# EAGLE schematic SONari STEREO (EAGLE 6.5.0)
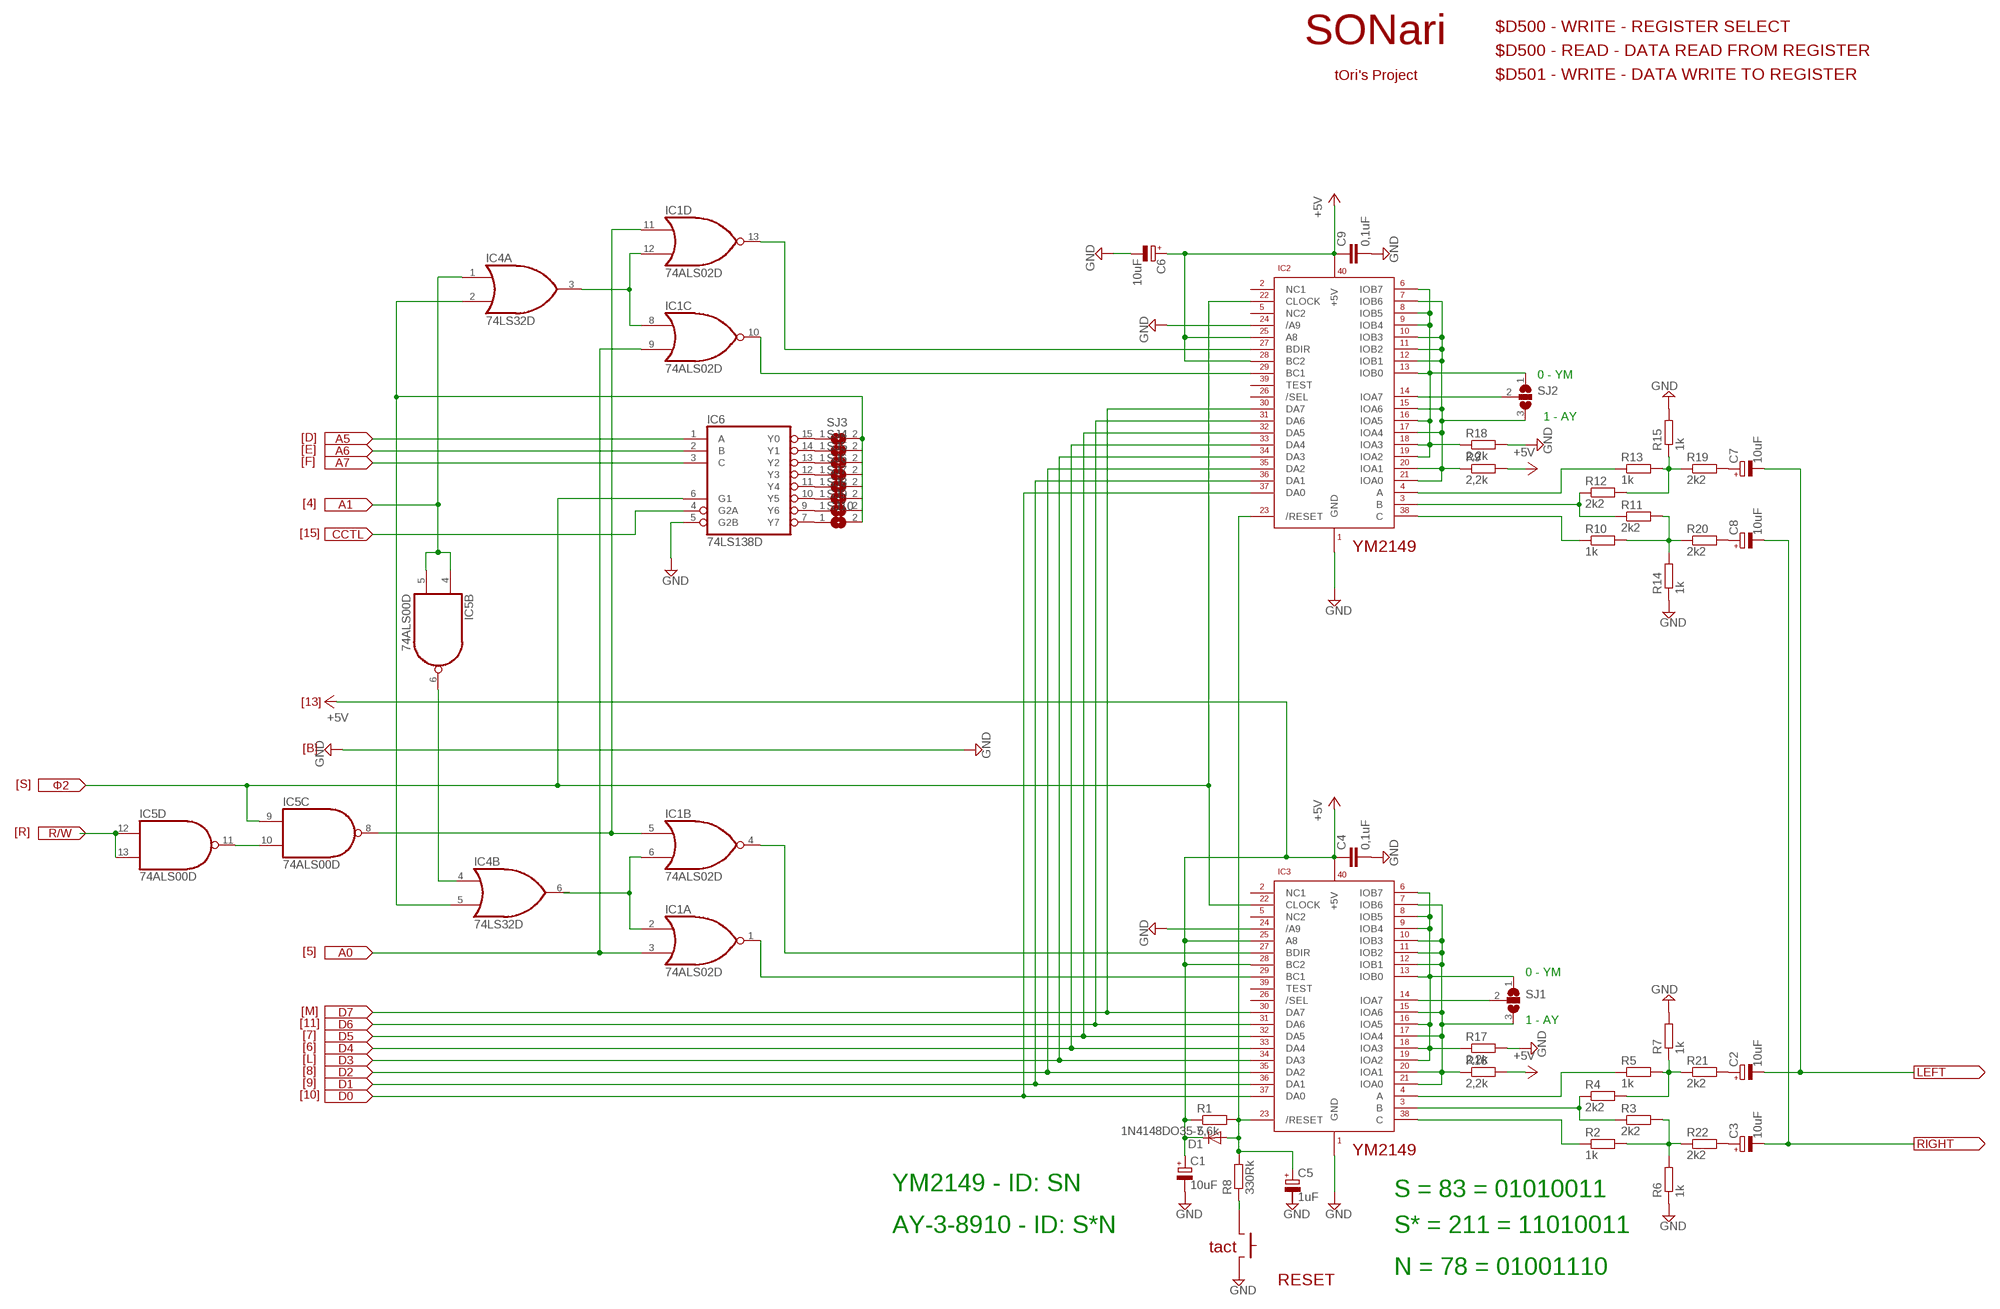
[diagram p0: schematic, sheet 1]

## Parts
C1  10uF  CPOL-EU085CS-1R  [085CS_1R]
C2  10uF  CPOL-EU085CS-1R  [085CS_1R]
C3  10uF  CPOL-EU085CS-1R  [085CS_1R]
C4  0,1uF  C-EUC0805  [C0805]
C5  1uF  CPOL-EU085CS-1R  [085CS_1R]
C6  10uF  CPOL-EU085CS-1R  [085CS_1R]
C7  10uF  CPOL-EU085CS-1R  [085CS_1R]
C8  10uF  CPOL-EU085CS-1R  [085CS_1R]
C9  0,1uF  C-EUC0805  [C0805]
D1  1N4148DO35-7  [DO35-7]
IC1  74ALS02D  [SO14]
IC2  YM2149  [YM2149]
IC3  YM2149  [YM2149]
IC4  74LS32D  [SO14]
IC5  74ALS00D  [SO14]
IC6  74LS138D  [SO16]
R1  5,6k  R-EU_R0805  [R0805]
R2  1k  R-EU_R0805  [R0805]
R3  2k2  R-EU_R0805  [R0805]
R4  2k2  R-EU_R0805  [R0805]
R5  1k  R-EU_R0805  [R0805]
R6  1k  R-EU_R0805  [R0805]
R7  1k  R-EU_R0805  [R0805]
R8  330Rk  R-EU_R0805  [R0805]
R9  2,2k  R-EU_R0805  [R0805]
R10  1k  R-EU_R0805  [R0805]
R11  2k2  R-EU_R0805  [R0805]
R12  2k2  R-EU_R0805  [R0805]
R13  1k  R-EU_R0805  [R0805]
R14  1k  R-EU_R0805  [R0805]
R15  1k  R-EU_R0805  [R0805]
R16  2,2k  R-EU_R0805  [R0805]
R17  2,2k  R-EU_R0805  [R0805]
R18  2,2k  R-EU_R0805  [R0805]
R19  2k2  R-EU_R0805  [R0805]
R20  2k2  R-EU_R0805  [R0805]
R21  2k2  R-EU_R0805  [R0805]
R22  2k2  R-EU_R0805  [R0805]
SJ1  SJ2W  [SJ_2]
SJ2  SJ2W  [SJ_2]
SJ3  SJ  [SJ]
SJ4  SJ  [SJ]
SJ5  SJ  [SJ]
SJ6  SJ  [SJ]
SJ7  SJ  [SJ]
SJ8  SJ  [SJ]
SJ9  SJ  [SJ]
SJ10  SJ  [SJ]

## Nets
+5V: C1.+ C6.+ D1.C IC2.P$25(A8) IC2.P$28(BC2) IC2.P$40(+5V) IC3.P$25(A8) IC3.P$28(BC2) IC3.P$40(+5V) R1.1 R9.2 R16.2
GND: C1.- C4.2 C6.- C9.2 IC2.P$1(GND) IC2.P$24(/A9) IC3.P$1(GND) IC3.P$24(/A9) IC6.5(G2B) R6.1 R7.2 R14.1 R15.2 R17.2 R18.2
N$1: IC1.1(A:O) IC3.P$29(BC1)
N$2: IC1.4(B:O) IC3.P$27(BDIR)
N$3: IC1.2(A:I0) IC1.6(B:I1)
N$4: IC1.5(B:I0) IC1.11(D:I0) IC5.8(C:O)
N$5: IC1.3(A:I1) IC1.9(C:I1)
N$6: IC2.P$31(DA6) IC2.P$33(DA4) IC2.P$34(DA3) IC2.P$36(DA1)
N$7: D1.A IC2.P$23(/RESET) IC3.P$23(/RESET) R1.2 R8.2
N$8: R8.1
N$10: IC1.10(C:O) IC2.P$29(BC1)
N$11: IC1.13(D:O) IC2.P$27(BDIR)
N$12: IC1.8(C:I0) IC1.12(D:I1) IC4.3(A:O)
N$13: IC3.P$3(B) R3.1 R4.1
N$14: IC3.P$4(A) R5.1
N$15: IC3.P$38(C) R2.1
N$16: R2.2 R3.2 R6.2 R22.1
N$17: R4.2 R5.2 R7.1 R21.1
N$18: C3.- C8.-
N$19: C2.- C7.-
N$20: IC5.12(D:I0) IC5.13(D:I1)
N$21: IC5.6(B:O)
N$22: IC2.P$30(DA7) IC2.P$32(DA5) IC2.P$35(DA2) IC2.P$37(DA0) IC3.P$30(DA7)
N$23: IC3.P$7(IOB6) IC3.P$10(IOB3) IC3.P$11(IOB2) IC3.P$12(IOB1) IC3.P$15(IOA6) IC3.P$17(IOA4) IC3.P$20(IOA1) IC3.P$21(IOA0) R16.1 SJ1.3
N$24: IC3.P$6(IOB7) IC3.P$8(IOB5) IC3.P$9(IOB4) IC3.P$13(IOB0) IC3.P$16(IOA5) IC3.P$18(IOA3) IC3.P$19(IOA2) R17.1 SJ1.1
N$25: IC2.P$3(B) R11.1 R12.1
N$26: IC2.P$4(A) R13.1
N$27: IC2.P$38(C) R10.1
N$28: R10.2 R11.2 R14.2 R20.1
N$29: R12.2 R13.2 R15.1 R19.1
N$30: C3.+ R22.2
N$31: C2.+ R21.2
N$32: IC3.P$14(IOA7) SJ1.2
N$33: IC2.P$7(IOB6) IC2.P$10(IOB3) IC2.P$11(IOB2) IC2.P$12(IOB1) IC2.P$15(IOA6) IC2.P$17(IOA4) IC2.P$20(IOA1) IC2.P$21(IOA0) R9.1 SJ2.3
N$34: IC2.P$14(IOA7) SJ2.2
N$35: IC2.P$6(IOB7) IC2.P$8(IOB5) IC2.P$9(IOB4) IC2.P$13(IOB0) IC2.P$16(IOA5) IC2.P$18(IOA3) IC2.P$19(IOA2) R18.1 SJ2.1
N$36: C7.+ R19.2
N$37: IC4.1(A:I0) IC5.4(B:I0) IC5.5(B:I1)
N$38: C8.+ R20.2
N$42: IC6.1(A)
N$43: IC6.3(C)
N$44: IC6.2(B)
N$46: IC6.4(G2A)
N$47: IC6.15(Y0) SJ3.1
N$48: IC6.14(Y1) SJ4.1
N$49: IC6.13(Y2) SJ5.1
N$50: IC6.12(Y3) SJ6.1
N$51: IC6.11(Y4) SJ7.1
N$52: IC6.10(Y5) SJ8.1
N$53: IC6.9(Y6) SJ9.1
N$54: IC6.7(Y7) SJ10.1
N$55: IC4.2(A:I1) IC4.5(B:I1) SJ3.2 SJ10.2
N$56: IC5.10(C:I1) IC5.11(D:O)
N$57: IC2.P$22(CLOCK) IC3.P$22(CLOCK) IC5.9(C:I0) IC6.6(G1)
Unconnected: C4.1 C5.+ C5.- C9.1 IC2.P$2(NC1) IC2.P$5(NC2) IC2.P$26(/SEL) IC2.P$39(TEST) IC3.P$2(NC1) IC3.P$5(NC2) IC3.P$26(/SEL) IC3.P$31(DA6) IC3.P$32(DA5) IC3.P$33(DA4) IC3.P$34(DA3) IC3.P$35(DA2) IC3.P$36(DA1) IC3.P$37(DA0) IC3.P$39(TEST) IC4.4(B:I0) IC4.6(B:O) IC4.8(C:O) IC4.9(C:I0) IC4.10(C:I1) IC4.11(D:O) IC4.12(D:I0) IC4.13(D:I1) IC5.1(A:I0) IC5.2(A:I1) IC5.3(A:O) SJ4.2 SJ5.2 SJ6.2 SJ7.2 SJ8.2 SJ9.2

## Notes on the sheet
- $D500 - WRITE - REGISTER SELECT
- SONari
- $D500 - READ - DATA READ FROM REGISTER
- tOri's Project | $D501 - WRITE - DATA WRITE TO REGISTER
- 0 - YM
- 1 - AY
- [D] | A5
- [E] | A6
- [F] | A7
- [4] | A1
- [15] | CCTL
- YM2149
- [13]
- [B]
- [S] | Φ2
- [R] | R/W
- [5] | A0
- 0 - YM
- [M] | D7
- [11] | 1 - AY
- D6
- [7] | D5
- [6] | D4
- [L] | D3
- [8] | D2 | LEFT
- [9] | D1
- [10] | D0
- RIGHT
- YM2149
- YM2149 - ID: SN | S = 83 = 01010011
- AY-3-8910 - ID: S*N | S* = 211 = 11010011
- tact
- N = 78 = 01001110
- RESET

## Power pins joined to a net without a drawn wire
GND: IC1.7(P:GND) IC4.7(P:GND) IC5.7(P:GND) IC6.8(GND)
VCC: IC1.14(P:VCC) IC4.14(P:VCC) IC5.14(P:VCC) IC6.16(VCC)

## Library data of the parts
C1-C3 C5-C8 = rcl:CPOL-EU: POLARIZED CAPACITOR, European symbol
C4 C9 = rcl:C-EU: CAPACITOR, European symbol
D1 = diode:1N4148: DIODE
IC1 = 74xx-us:74*02: Quad 2-input NOR gate
IC2 IC3 = YM2149:YM2149
IC4 = 74xx-us:74*32: Quad 2-input OR gate
IC5 = 74xx-us:74*00: Quad 2-input NAND gate
IC6 = 74xx-us:74*138: 3-line to 8-line DECODER/DEMULTIPLEXER
R1-R22 = rcl:R-EU_: RESISTOR, European symbol
SJ1 SJ2 = jumper:SJ2W: SMD solder JUMPER
SJ3-SJ10 = jumper:SJ: SMD solder JUMPER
